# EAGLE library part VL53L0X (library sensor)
VL53L0X distance sensor
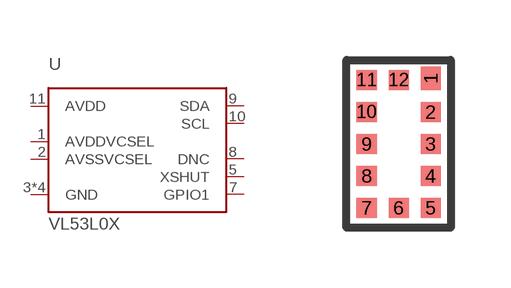
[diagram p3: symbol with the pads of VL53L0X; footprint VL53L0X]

Designator prefix U

## VL53L0X  [VL53L0X]
1  AVDDVCSEL
2  AVSSVCSEL
3  GND
4  GND
5  XSHUT
6  GND
7  GPIO1
8  DNC
9  SDA
10  SCL
11  AVDD
12  GND

## Footprint VL53L0X (pad centres in mm)
smd 0.5 x 0.58: 1 0.8,1.64
smd 0.5 x 0.5: 2 0.8,0.8; 3 0.8,0; 4 0.8,-0.8; 5 0.8,-1.6; 6 0,-1.6; 7 -0.8,-1.6; 8 -0.8,-0.8; 9 -0.8,0; 10 -0.8,0.8; 11 -0.8,1.6; 12 0,1.6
